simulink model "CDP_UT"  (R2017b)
settings: Solver=FixedStepDiscrete  StartTime=0.0  StopTime=10.0  FixedStep=0.01  RelTol=1e-3  EnableMultiTasking=on
undefined symbols (not defined in the file): ASWTYPE_FALSE, ASWTYPE_TRUE, CaCDP_CellTempNTCVoltTable_mV, CaCDP_CellTempTable_C, CaCDP_CMUPCBTempNTCVoltTable_mV, CaCDP_CMUPCBTempTable_C, CbCDP_DiffBusbarTempStateCheck_flg, CbCDP_DiffCellTempStateCheck_flg, CbCDP_DiffCellVoltStateCheck_flg, CbCDP_IgnorUpdateVld_flg, CbCDP_MaxBusbarTempStateCheck_flg, CbCDP_MaxCellTempStateCheck_flg, CbCDP_MaxCellVoltStateCheck_flg, CbCDP_MinBusbarTempStateCheck_flg, CbCDP_MinCellTempStateCheck_flg, CbCDP_MinCellVoltStateCheck_flg, CcCDP_AFETempConfig_numb, CcCDP_AFETempFltThd_C, CcCDP_AFETempFltThdHys_C, CcCDP_BusbarTempRngFltHiThrd_C, CcCDP_BusbarTempRngFltLowThrd_C, CcCDP_CellDiffFltLevel1_mV, CcCDP_CellDiffFltLevel2_mV, CcCDP_CellDiffFltLevel3_mV, CcCDP_CellTempLowerLimit_C, CcCDP_CellTempRngFltHiThrd_C, CcCDP_CellTempRngFltLowThrd_C, CcCDP_CellTempUpperLimit_C, CcCDP_CellVoltConfig_numb, CcCDP_CellVoltLowerLimit_mV, CcCDP_CellVoltRngHiThrd_mV, CcCDP_CellVoltRngLowThrd_mV, CcCDP_CellVoltUpdateThrd_numb, CcCDP_CellVoltUpperLimit_mV, CcCDP_ChrgMaxCellTempFltLv1Thrd_C, CcCDP_ChrgMaxCellTempFltLv2Thrd_C, CcCDP_ChrgMaxCellTempFltLv3Thrd_C, CcCDP_ChrgMaxCellTempReturnDiff_C, CcCDP_ChrgMinCellTempFltLv1Thrd_C, CcCDP_ChrgMinCellTempFltLv2Thrd_C, CcCDP_ChrgMinCellTempFltLv3Thrd_C, CcCDP_ChrgMinCellTempReturnDiff_C, CcCDP_CMUPCBTempConfig_numb, CcCDP_CMUPCBTempFltThd_C, CcCDP_CMUPCBTempFltThdHys_C, CcCDP_DiffBusbarTempFltLevel1Thrd_C, CcCDP_DiffBusbarTempFltLevel2Thrd_C, CcCDP_DiffBusbarTempReturnDifference_C, CcCDP_DiffCellTempFltLevel1Thrd_C, CcCDP_DiffCellTempFltLevel2Thrd_C, CcCDP_DiffCellTempReturnDifference_C, CcCDP_DiffCellVoltReturnDifference_mV, CcCDP_DiffVoltCheckMaxCellTempCondition_C, CcCDP_DiffVoltCheckMaxCellVoltCondition_mV, CcCDP_DiffVoltCheckMinCellTempCondition_C, CcCDP_DiffVoltCheckMinCellVoltCondition_mV, CcCDP_DiffVoltCheckPackCurrCondition_A, CcCDP_MaxAFETempIniVal_C, CcCDP_MaxBusbarTempFltLevel1Thrd_C, CcCDP_MaxBusbarTempFltLevel2Thrd_C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
libraries: AIWAYS_Powertrain_BMS_lib x148, simulink x8
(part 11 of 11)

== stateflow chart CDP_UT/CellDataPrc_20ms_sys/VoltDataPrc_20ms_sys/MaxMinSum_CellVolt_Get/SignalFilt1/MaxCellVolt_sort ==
  state sort
    (default) -> (junction 6) : /*Input value sort from big to small*/
    sort -> (junction 6)
    (junction 6) -> (junction 8) : {i = 0;temp = 0;}
    (junction 8) -> (junction 12) : [i < Input_dim]
    (junction 12) -> (junction 14) : {Output_Value[i] = Input_Value[i];}
    (junction 14) -> (junction 8) : {i++;}
    (junction 8) -> (junction 17) : {i=0;}
    (junction 25) -> (junction 31) : [Output_Value[j] > temp]
    (junction 17) -> (junction 19) : [i < Input_dim]
    (junction 21) -> (junction 25) : [j < Input_dim]
    (junction 19) -> (junction 21) : {temp = 0;Output_index[i] = 0;j = 0;}
    (junction 25) -> (junction 34)
    (junction 31) -> (junction 32) : {temp = Output_Value[j]; Output_index[i] = j;}
    (junction 38) -> (junction 17) : {i++;}
    (junction 34) -> (junction 21) : {j++;}
    (junction 21) -> (junction 38) : {Output_Value[Output_index[i]] = 0;}
    (junction 17) -> (junction 41) : {i= 0;}
    (junction 32) -> (junction 34)
    (junction 41) -> (junction 43) : [i < Input_dim]
    (junction 43) -> (junction 45) : {Output_Value[i] = Input_Value[Output_index[i]];}
    (junction 45) -> (junction 41) : {i++;}
    (junction 41) -> (junction 48)
  (default) -> sort
  data: Input_Value input uint16; Input_dim input uint8; Output_Value output single; i local uint8; temp local single; j local uint8; Output_index output uint16
